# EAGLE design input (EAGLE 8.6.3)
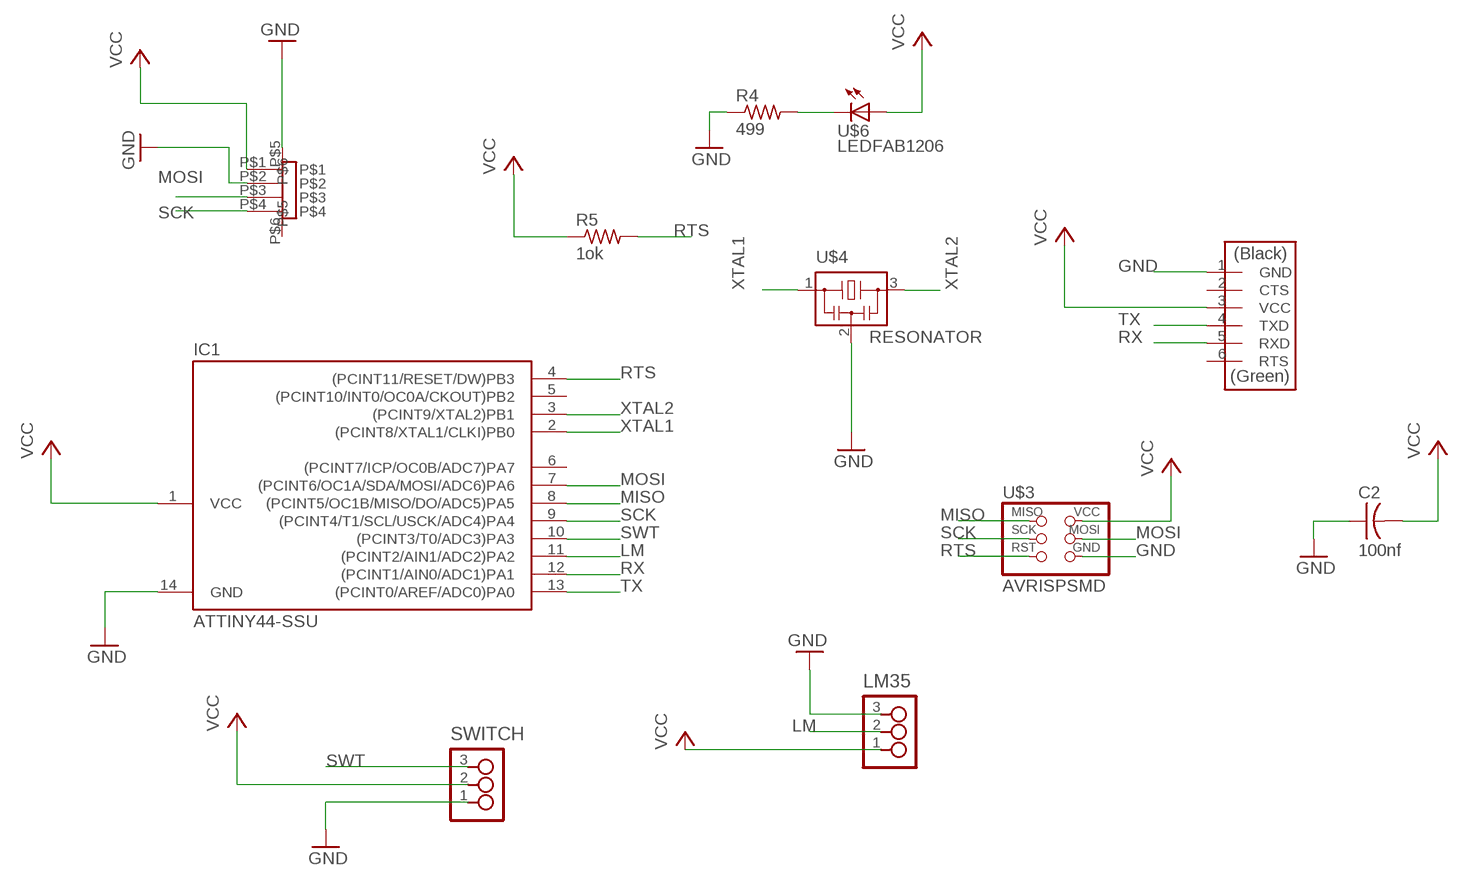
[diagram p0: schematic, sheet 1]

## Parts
C2  100nf  CAP-US1206K  [C1206K]
FTDI  FTDI-SMD-HEADER  [1X06SMD]
IC1  ATTINY44-SSU  [SOIC14]
LM35  3_PIN_HEADERHEADER  [SMT_PINS_3]
R4  499  RES-US1206FAB  [R1206FAB]
R5  1ok  RES-US1206FAB  [R1206FAB]
SWITCH  3_PIN_HEADERHEADER  [SMT_PINS_3]
U$3  AVRISPSMD  [2X03SMD]
U$4  RESONATOR  [EFOBM]
U$6  LEDFAB1206  [LED1206FAB]
U$9  PHP4_SM4  [PH4P_SM4]

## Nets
GND: C2.1 FTDI.1(GND) IC1.14(GND) LM35.3 R4.1 SWITCH.1 U$3.6(GND) U$4.2 U$9.P$2 U$9.P$5
LM: IC1.11((PCINT2/AIN1/ADC2)PA2) LM35.2
MISO: IC1.8((PCINT5/OC1B/MISO/DO/ADC5)PA5) U$3.1(MISO)
MOSI: IC1.7((PCINT6/OC1A/SDA/MOSI/ADC6)PA6) U$3.4(MOSI) U$9.P$3
N$7: R4.2 U$6.2(C)
RTS: IC1.4((PCINT11/RESET/DW)PB3) R5.2 U$3.5(RST)
RX: FTDI.5(RXD) IC1.12((PCINT1/AIN0/ADC1)PA1)
SCK: IC1.9((PCINT4/T1/SCL/USCK/ADC4)PA4) U$3.3(SCK) U$9.P$4
SWT: IC1.10((PCINT3/T0/ADC3)PA3) SWITCH.3
TX: FTDI.4(TXD) IC1.13((PCINT0/AREF/ADC0)PA0)
VCC: C2.2 FTDI.3(VCC) IC1.1(VCC) LM35.1 R5.1 SWITCH.2 U$3.2(VCC) U$6.1(A) U$9.P$1
XTAL1: IC1.2((PCINT8/XTAL1/CLKI)PB0) U$4.1
XTAL2: IC1.3((PCINT9/XTAL2)PB1) U$4.3
Unconnected: FTDI.2(CTS) FTDI.6(RTS) IC1.5((PCINT10/INT0/OC0A/CKOUT)PB2) IC1.6((PCINT7/ICP/OC0B/ADC7)PA7) U$9.P$6

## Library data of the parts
C2 = fab:CAP-US
FTDI = fab:FTDI-SMD-HEADER
IC1 = fab:ATTINY44
LM35 SWITCH = FabLab:3_PIN_HEADER: 3 SMT pin pads
R4 R5 = fab:RES-US: Resistor (US Symbol)
U$3 = fab:AVRISP
U$4 = fab:RESONATOR
U$6 = fab:LED: LED
U$9 = jst_ph_topo:PHP4_SM4

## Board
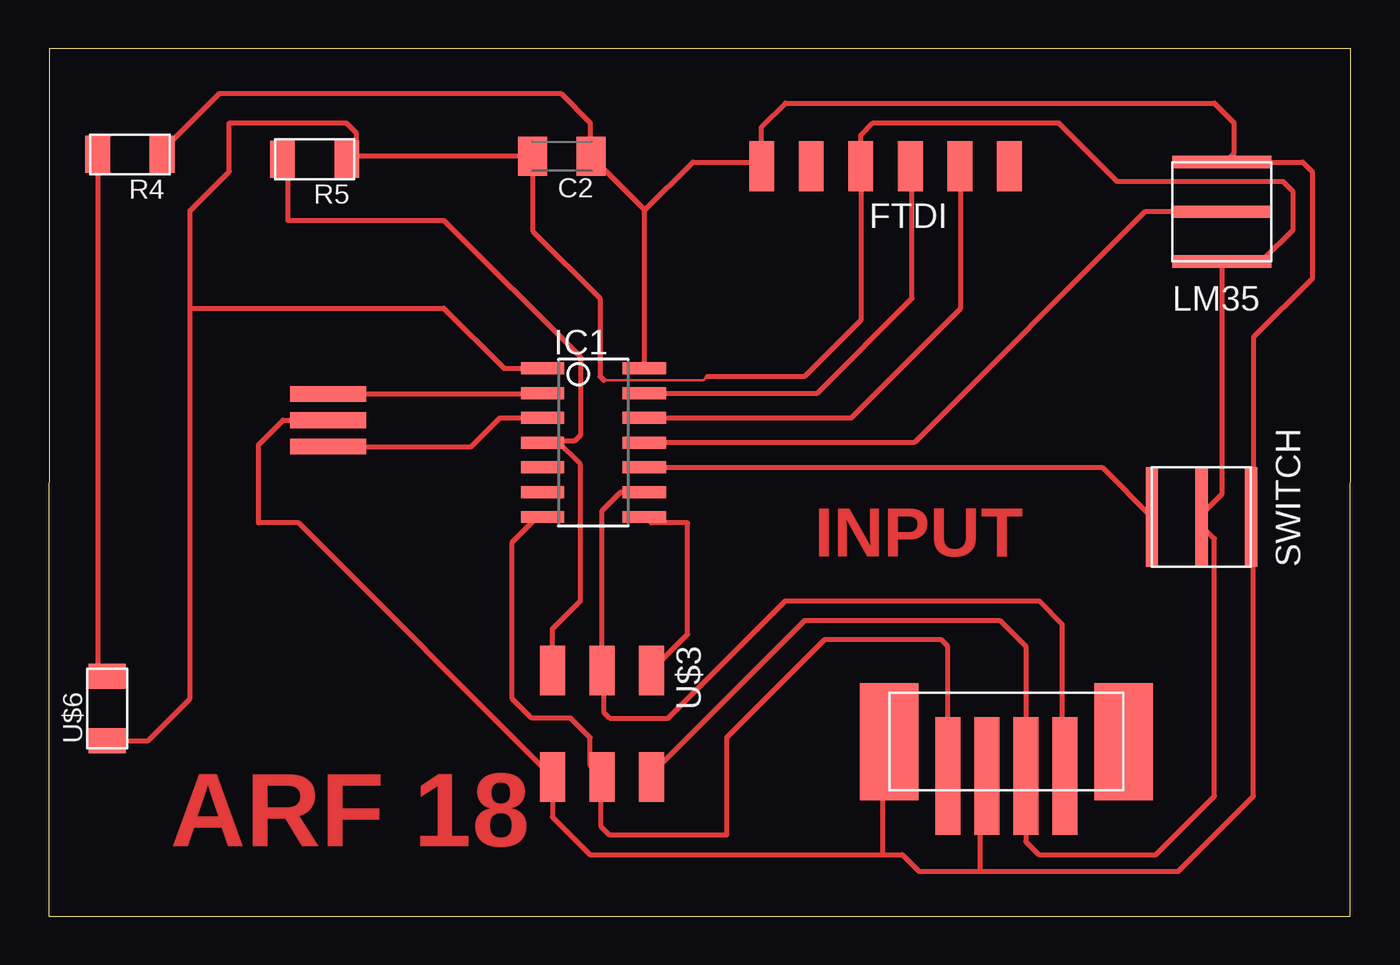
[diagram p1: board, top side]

Size 66.73 x 44.43 mm. Coordinates in mm from the lower left corner, seen from the top.
Outline: 0,0 66.7,0 66.73,44.43 0.03,44.43 0,0
Copper layers (1*16): Top 0.35mm / dielectric 0.5mm / Bottom 0.35mm
Design rules "default *": minimum track width 6mil, minimum drill 0.35mm, track to track 6mil, track to pad 6mil, pad to pad 6mil, via to via 6mil, smd to smd 6mil, copper to edge 40mil, drill to drill 6mil, minimum pad ring 10mil, minimum via ring 8mil, stop-mask expansion 4mil, vias tented up to drill 0mil, thermal gap 10mil

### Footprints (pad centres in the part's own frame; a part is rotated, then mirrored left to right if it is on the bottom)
C1206K = smd 1.5 x 2: 1 -1.5,0; 2 1.5,0
1X06SMD = smd 2.54 x 1.27: 1 0,6.35; 2 0,3.81; 3 0,1.27; 4 0,-1.27; 5 0,-3.81; 6 0,-6.35
SOIC14 = smd 0.61 x 2.21: 1 -3.81,-2.603; 2 -2.54,-2.603; 3 -1.27,-2.603; 4 0,-2.603; 5 1.27,-2.603; 6 2.54,-2.603; 7 3.81,-2.603; 8 3.81,2.603; 9 2.54,2.603; 10 1.27,2.603; 11 0,2.603; 12 -1.27,2.603; 13 -2.54,2.603; 14 -3.81,2.603
SMT_PINS_3 = smd 5.08 x 0.635: 1 0,0; 2 0,2.54; 3 0,5.08
R1206FAB = smd 1.27 x 1.905: 1 -1.651,0; 2 1.651,0
2X03SMD = smd 2.54 x 1.27: 1 -2.54,2.54; 2 2.92,2.54; 3 -2.54,0; 4 2.92,0; 5 -2.54,-2.54; 6 2.92,-2.54
EFOBM = smd 0.8 x 3.9: 1 -1.35,0; 2 0,0; 3 1.35,0
LED1206FAB = smd 1.27 x 1.905: 1 -1.651,0; 2 1.651,0
PH4P_SM4 = smd 6 x 1.27: P$1 2,2; P$2 2,4; P$3 2,6; P$4 2,0 | smd 6 x 3: P$5 3.75,9; P$6 3.75,-3

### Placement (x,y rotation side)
C2  26.3,38.92 180 top
FTDI  42.89,38.41 90 top
IC1  27.92,24.25 270 top
LM35  60.12,33.54 0 top
R4  4.16,39.02 180 top
R5  13.63,38.77 180 top
SWITCH  61.62,20.44 90 top
U$3  28.36,10.04 270 top
U$4  14.32,25.4 270 top
U$6  3,10.63 90 top
U$9  52.08,5.17 90 top

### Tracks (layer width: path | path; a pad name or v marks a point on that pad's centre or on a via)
GND
  Top 0.152: 26.18,7.02 25.87,7.02 U$3.6 25.72,7.17 | 42.94,8.85 U$9.P$5 | 61.38,38.57 60.25,38.57 60.16,38.57 LM35.3 60.01,38.72 | 61.69,20.58 SWITCH.1 | 5.91,39.02 R4.1 | 27.7,39.02 C2.1 27.85,38.87 | 30.45,28.2 IC1.14 | 36.39,38.26 FTDI.1 36.76,38.63
  Top 0.254: U$4.2 12.01,25.4 10.75,24.14 10.75,20.14 12.8,20.14 U$3.6 25.82,5.07 27.75,3.14 42.75,3.14 | 42.75,3.14 42.75,8.65 42.94,8.85 | 42.75,3.14 43.75,3.14 44.6,2.29 47.75,2.29 | 61.75,20.31 SWITCH.1 | 47.75,2.29 57.89,2.29 61.75,6.14 61.75,20.31 | 47.75,2.29 47.75,6.84 U$9.P$2 | 30.52,36.14 30.52,36.2 C2.1 27.75,38.97 27.75,40.64 26.25,42.14 8.75,42.14 5.81,39.2 R4.1 | 30.52,36.14 IC1.14 | 30.52,36.14 33.01,38.63 36.76,38.63 | FTDI.1 36.54,40.43 37.75,41.64 59.75,41.64 60.75,40.64 60.75,39.07 60.25,38.57 | LM35.3 64.27,38.62 64.75,38.14 64.75,32.64 61.75,29.64 61.75,20.31
LM
  Top 0.152: 59.25,35.98 60.01,35.98 LM35.2 | 30.6,24.39 IC1.11
  Top 0.254: LM35.2 56.19,36.08 44.36,24.25 IC1.11
MISO
  Top 0.152: 30.6,12.81 30.75,12.66 U$3.1 | 30.6,20.43 IC1.8
  Top 0.254: U$3.1 32.75,14.43 32.75,20.14 30.89,20.14 30.6,20.43
MOSI
  Top 0.152: 25.26,20.43 IC1.7 | 28.31,7.17 U$3.4 | 45.99,7.33 U$9.P$3
  Top 0.254: U$9.P$3 46.08,13.81 45.75,14.14 39.75,14.14 34.75,9.14 34.75,4.14 28.75,4.14 28.31,4.58 28.31,7.17 | U$3.4 27.75,7.73 27.75,9.14 26.75,10.14 24.75,10.14 23.75,11.14 23.75,19.14 25.03,20.43 25.26,20.43
N$7
  Top 0.152: 2.56,12.66 2.86,12.35 U$6.2 | 2.56,38.87 R4.2
  Top 0.254: R4.2 2.5,12.71 2.86,12.35
RTS
  Top 0.152: 12.01,38.72 R5.2 | 25.87,12.66 U$3.5 | 25.42,24.39 26.03,24.39 25.71,24.33 IC1.4 25.42,24.39
  Top 0.254: U$3.5 25.82,14.71 27.25,16.14 27.25,23.14 26.06,24.33 | 26.06,24.33 25.71,24.33 | R5.2 12.25,38.5 12.25,35.64 20.25,35.64 27.25,28.64 27.25,24.64 26.93,24.33 26.06,24.33
RX
  Top 0.152: 30.6,25.61 IC1.12 | 46.6,38.26 FTDI.5
  Top 0.254: IC1.12 41.13,25.52 46.75,31.14 46.75,38.36 FTDI.5
SCK
  Top 0.152: 29.99,21.65 30.45,21.65 IC1.9 | 28.46,13.14 28.46,12.66 U$3.3 28.46,12.51 | 51.93,9.31 51.93,7.33 U$9.P$4
  Top 0.254: 28.75,12.38 28.46,12.66 | 28.46,13.14 28.46,10.43 28.75,10.14 31.75,10.14 37.75,16.14 50.75,16.14 51.93,14.96 51.93,7.33 | U$3.3 28.36,20.75 29.32,21.71 IC1.9
SWT
  Top 0.152: 30.6,22.87 IC1.10 | 56.51,20.58 SWITCH.3
  Top 0.254: IC1.10 54,22.98 SWITCH.3
TX
  Top 0.152: 30.6,26.83 IC1.13 | 44.01,38.26 FTDI.4
  Top 0.254: IC1.13 39.4,26.79 44.25,31.64 44.25,38.32 FTDI.4
VCC
  Top 0.127: 28.45,27.44 33.54,27.44 33.75,27.64
  Top 0.152: 3.01,9 U$6.1 | 15.21,38.87 R5.1 15.36,38.87 | 24.65,38.87 C2.2 24.81,38.87 | 25.26,28.2 IC1.1 | 49.95,9.31 49.95,7.33 U$9.P$1 50.1,7.17 50.1,5.04 | 30.9,7.17 U$3.2 | U$3.2 | 60.92,33.69 60.16,33.69 LM35.1 60.01,33.54 | 59.1,20.58 SWITCH.2 58.94,20.43 58.94,20.14 58.94,19.67 | 41.57,37.35 41.57,38.26 FTDI.3
  Top 0.254: 58.94,20.14 59.75,19.34 59.75,6.14 56.75,3.14 50.75,3.14 50.08,3.81 U$9.P$1 50.08,13.81 48.75,15.14 38.75,15.14 30.9,7.29 U$3.2 | 59.1,20.58 60.12,21.6 LM35.1 60.22,33.64 62.25,33.64 63.75,35.14 63.75,37.14 63.25,37.64 54.75,37.64 51.75,40.64 42.25,40.64 41.62,40.01 FTDI.3 41.62,30.51 38.75,27.64 33.75,27.64 | 15.75,38.92 C2.2 24.8,35.09 28.25,31.64 28.25,27.64 28.45,27.44 | 15.75,38.92 15.43,38.92 R5.1 | U$6.1 5.08,8.98 7.25,11.14 7.25,31.14 | 7.25,31.14 7.25,36.14 9.25,38.14 9.25,40.64 15.25,40.64 15.75,40.14 15.75,38.92 | 7.25,31.14 20.25,31.14 23.33,28.06 IC1.1
XTAL1
  Top 0.152: 25.26,26.68 IC1.2
  Top 0.254: U$4.1 25.27,26.75 IC1.2
XTAL2
  Top 0.254: U$4.3 21.66,24.05 23.13,25.52 IC1.3

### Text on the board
Top: INPUT | ARF 18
